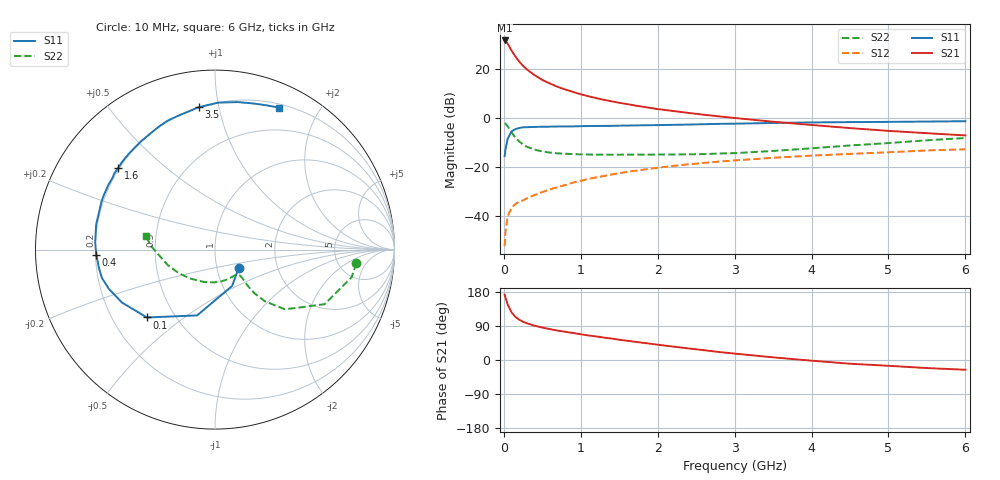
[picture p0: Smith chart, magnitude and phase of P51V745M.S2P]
! SIEMENS Small Signal Semiconductors
! BFP183
! Si NPN RF Bipolar Junction Transistor in SOT143
! VCE = 1.75 V  IC = 45 mA
! Common Emitter S-Parameters:  March  1996
# GHz  S  MA  R  50
!  f  S11  S21  S12  S22
! GHz  MAG  ANG  MAG  ANG  MAG  ANG  MAG  ANG
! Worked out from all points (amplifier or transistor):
!   36 points, 10 MHz to 6 GHz, reference 50 ohm
!   highest |S21| = 31.8 dB at 10 MHz (marker M1)
!   |S21| within 3 dB of that: start of sweep to 80.08 MHz
!   unconditionally stable (mu >= 1): start of sweep to 21.31 MHz; 244 MHz to end of sweep
!   at 250 MHz: K = 1.02, MAG = 26.8 dB, |S12| = -33.6 dB
!   at 1.4 GHz: K = 1.57, MAG = 10.5 dB, |S12| = -23.1 dB
!   at 6 GHz: K = 1.21, MAG = 0.1 dB, |S12| = -12.7 dB
!   S11 on the Smith chart (normalised r, x): 10 MHz: 1.27, -0.27; 100 MHz: 0.35, -0.37; 400 MHz: 0.20, -0.02; 1.6 GHz: 0.20, +0.35; 3.5 GHz: 0.20, +0.87; 6 GHz: 0.24, +1.52
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0.01  0.1674 -38.2  39.01 172.7  0.0024 72.8  0.7917 -5.5
0.02  0.2241 -64.9  38.31 165.6  0.0046 73.6  0.7763 -11.5
0.05  0.3799 -105.2  33.51 146.3  0.0099 66.3  0.6819 -26.5
0.1  0.5358 -135.1  24.3 125.7  0.0146 50.1  0.5124 -40.5
0.15  0.5962 -150.3  18.26 113.7  0.0175 47.3  0.4003 -46.0
0.2  0.6303 -159.6  14.4 106.2  0.0195 47.0  0.3327 -47.8
0.25  0.6497 -166.0  11.78 100.8  0.0208 48.0  0.2895 -48.0
0.3  0.6545 -170.7  9.956 96.8  0.023 49.7  0.26 -47.6
0.4  0.6621 -177.6  7.589 90.4  0.0267 52.8  0.2269 -46.5
0.5  0.6687 176.6  6.079 85.6  0.0307 54.3  0.2087 -46.0
0.6  0.6711 172.2  5.116 81.4  0.035 57.5  0.1973 -46.2
0.7  0.6768 168.0  4.373 77.6  0.0389 58.7  0.1907 -46.8
0.9  0.6797 161.3  3.442 71.3  0.048 59.8  0.1844 -49.4
1.1  0.6899 154.1  2.814 64.8  0.0572 59.6  0.1805 -53.2
1.3  0.6956 148.5  2.376 59.2  0.0655 59.5  0.1794 -58.0
1.6  0.7056 139.7  1.944 50.9  0.0792 57.7  0.1795 -65.6
2.2  0.7306 124.3  1.404 35.4  0.1055 52.4  0.1805 -84.6
2.8  0.7651 110.2  1.088 21.0  0.1292 46.1  0.1889 -106.0
3.5  0.7981 96.6  0.846 7.0  0.1546 39.1  0.2132 -131.1
4.5  0.8315 81.3  0.627 -9.8  0.1858 28.9  0.2762 -161.6
5.5  0.8532 70.5  0.493 -21.3  0.2186 19.7  0.353 177.5
6  0.8671 65.9  0.444 -25.7  0.2312 14.6  0.3933 168.9
